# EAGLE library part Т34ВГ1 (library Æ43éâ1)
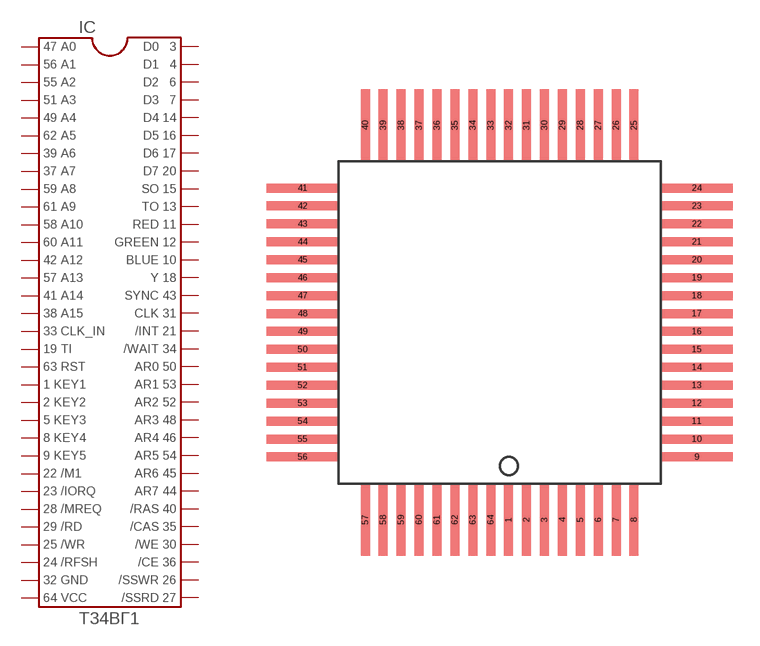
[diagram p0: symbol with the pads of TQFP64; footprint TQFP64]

Designator prefix IC

## Т34ВГ1  [TQFP64]
1  1  pas
2  2  pas
3  3  pas
4  4  pas
5  5  pas
6  6  pas
7  7  pas
8  8  pas
9  9  pas
10  10  pas
11  11  pas
12  12  pas
13  13  pas
14  14  pas
15  15  pas
16  16  pas
17  17  pas
18  18  pas
19  19  pas
20  20  pas
21  21  pas
22  22  pas
23  23  pas
24  24  pas
25  25  pas
26  26  pas
27  27  pas
28  28  pas
29  29  pas
30  30  pas
31  31  pas
32  32  pas
33  33  pas
34  34  pas
35  35  pas
36  36  pas
37  37  pas
38  38  pas
39  39  pas
40  40  pas
41  41  pas
42  42  pas
43  43  pas
44  44  pas
45  45  pas
46  46  pas
47  47  pas
48  48  pas
49  49  pas
50  50  pas
51  51  pas
52  52  pas
53  53  pas
54  54  pas
55  55  pas
56  56  pas
57  57  pas
58  58  pas
59  59  pas
60  60  pas
61  61  pas
62  62  pas
63  63  pas
64  64  pas

## Footprint TQFP64 (pad centres in mm)
Thin Plasic Quad Flat Package Updated from atml.lbr 17.01.2005 alf@cadsoft.de
smd 0.5 x 4: 1 -1.5,-13; 2 -0.5,-13; 3 0.5,-13; 4 1.5,-13; 5 2.5,-13; 6 3.5,-13; 7 4.5,-13; 8 5.5,-13; 25 5.5,9; 26 4.5,9; 27 3.5,9; 28 2.5,9; 29 1.5,9; 30 0.5,9; 31 -0.5,9; 32 -1.5,9; 33 -2.5,9; 34 -3.5,9; 35 -4.5,9; 36 -5.5,9; 37 -6.5,9; 38 -7.5,9; 39 -8.5,9; 40 -9.5,9; 57 -9.5,-13; 58 -8.5,-13; 59 -7.5,-13; 60 -6.5,-13; 61 -5.5,-13; 62 -4.5,-13; 63 -3.5,-13; 64 -2.5,-13
smd 4 x 0.5: 9 9,-9.5; 10 9,-8.5; 11 9,-7.5; 12 9,-6.5; 13 9,-5.5; 14 9,-4.5; 15 9,-3.5; 16 9,-2.5; 17 9,-1.5; 18 9,-0.5; 19 9,0.5; 20 9,1.5; 21 9,2.5; 22 9,3.5; 23 9,4.5; 24 9,5.5; 41 -13,5.5; 42 -13,4.5; 43 -13,3.5; 44 -13,2.5; 45 -13,1.5; 46 -13,0.5; 47 -13,-0.5; 48 -13,-1.5; 49 -13,-2.5; 50 -13,-3.5; 51 -13,-4.5; 52 -13,-5.5; 53 -13,-6.5; 54 -13,-7.5; 55 -13,-8.5; 56 -13,-9.5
